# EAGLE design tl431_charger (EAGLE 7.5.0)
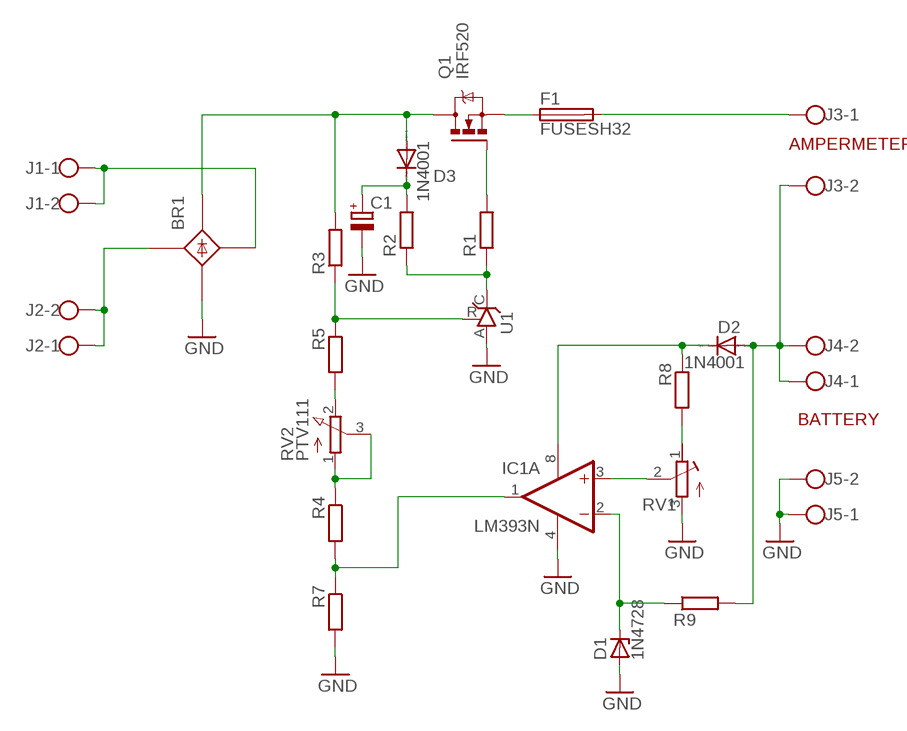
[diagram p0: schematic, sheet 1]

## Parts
BR1  B25A-  [B25A-]
C1  CPOL-EUE2.5-7  [E2,5-7]
D1  1N4728  [DO41Z10]
D2  1N4001  1N4004  [DO41-10]
D3  1N4001  1N4004  [DO41-10]
F1  FUSESH32  [SH32]
IC1  LM393N  [DIL08]
J1  W237-102  [W237-102]
J2  W237-102  [W237-102]
J3  W237-102  [W237-102]
J4  W237-102  [W237-102]
J5  W237-102  [W237-102]
Q1  IRF520  [TO220BV]
R1  R-EU_0207/10  [0207/10]
R2  R-EU_0207/10  [0207/10]
R3  R-EU_0207/10  [0207/10]
R4  R-EU_0207/10  [0207/10]
R5  R-EU_0207/10  [0207/10]
R7  R-EU_0207/10  [0207/10]
R8  R-EU_0207/10  [0207/10]
R9  R-EU_0207/10  [0207/10]
RV1  R-TRIMM-3386-F  [R-TRIMM-3386F]
RV2  PTV111  [PTV111]
U1  TL431CLP  [TO92-CLP]

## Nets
GND: BR1.-1(-) C1.- D1.A IC1.4(P:V-) J5.1 J5.2 R7.2 RV1.3(E) U1.A
N$1: IC1.1(A:OUT) R4.2 R7.1
N$2: Q1.G R1.2
N$3: F1.1A Q1.S
N$4: BR1.+1(+) D3.A Q1.D R3.2
N$5: C1.+ D3.C R2.2
N$6: R1.1 R2.1 U1.C
N$7: R5.2 RV2.2(E)
N$8: R3.1 R5.1 U1.R
N$9: R4.1 RV2.1(A) RV2.3(S)
N$10: IC1.3(A:+IN) RV1.2(S)
N$11: D1.C IC1.2(A:-IN) R9.1
N$12: BR1.AC1-(AC1) J2.1 J2.2
N$13: BR1.AC2-(AC2) J1.1 J1.2
N$14: R8.2 RV1.1(A)
N$15: D2.C IC1.8(P:V+) R8.1
N$16: D2.A J3.2 J4.1 J4.2 R9.2
N$17: F1.2A J3.1
Unconnected: BR1.+ BR1.- BR1.AC1 BR1.AC2 IC1.5(B:+IN) IC1.6(B:-IN) IC1.7(B:OUT)

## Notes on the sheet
- AMPERMETER
- BATTERY

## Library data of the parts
BR1 = rectifier:B25A-: RECTIFIER 25-A bridge
C1 = rcl:CPOL-EU: POLARIZED CAPACITOR, European symbol
D1 = diode:1N4728: Z DIODE
D2 D3 = diode:1N4004: DIODE
F1 = fuse:FUSE: Fuse; OC_FARNELL: unknown; OC_NEWARK: unknown
IC1 = linear:LM393: COMPARATOR
J1-J5 = con-wago-500:W237-102: WAGO SCREW CLAMP; MPN: 237-102; OC_FARNELL: unknown; OC_NEWARK: 70K9898
Q1 = transistor-power:IRF520: HEXFET Power MOSFET
R1-R5 R7-R9 = rcl:R-EU_: RESISTOR, European symbol
RV1 = rcl:R-TRIMM-3386-F
RV2 = pot:PTV111
U1 = v-reg:TL431CLP: VOLTAGE REGULATOR

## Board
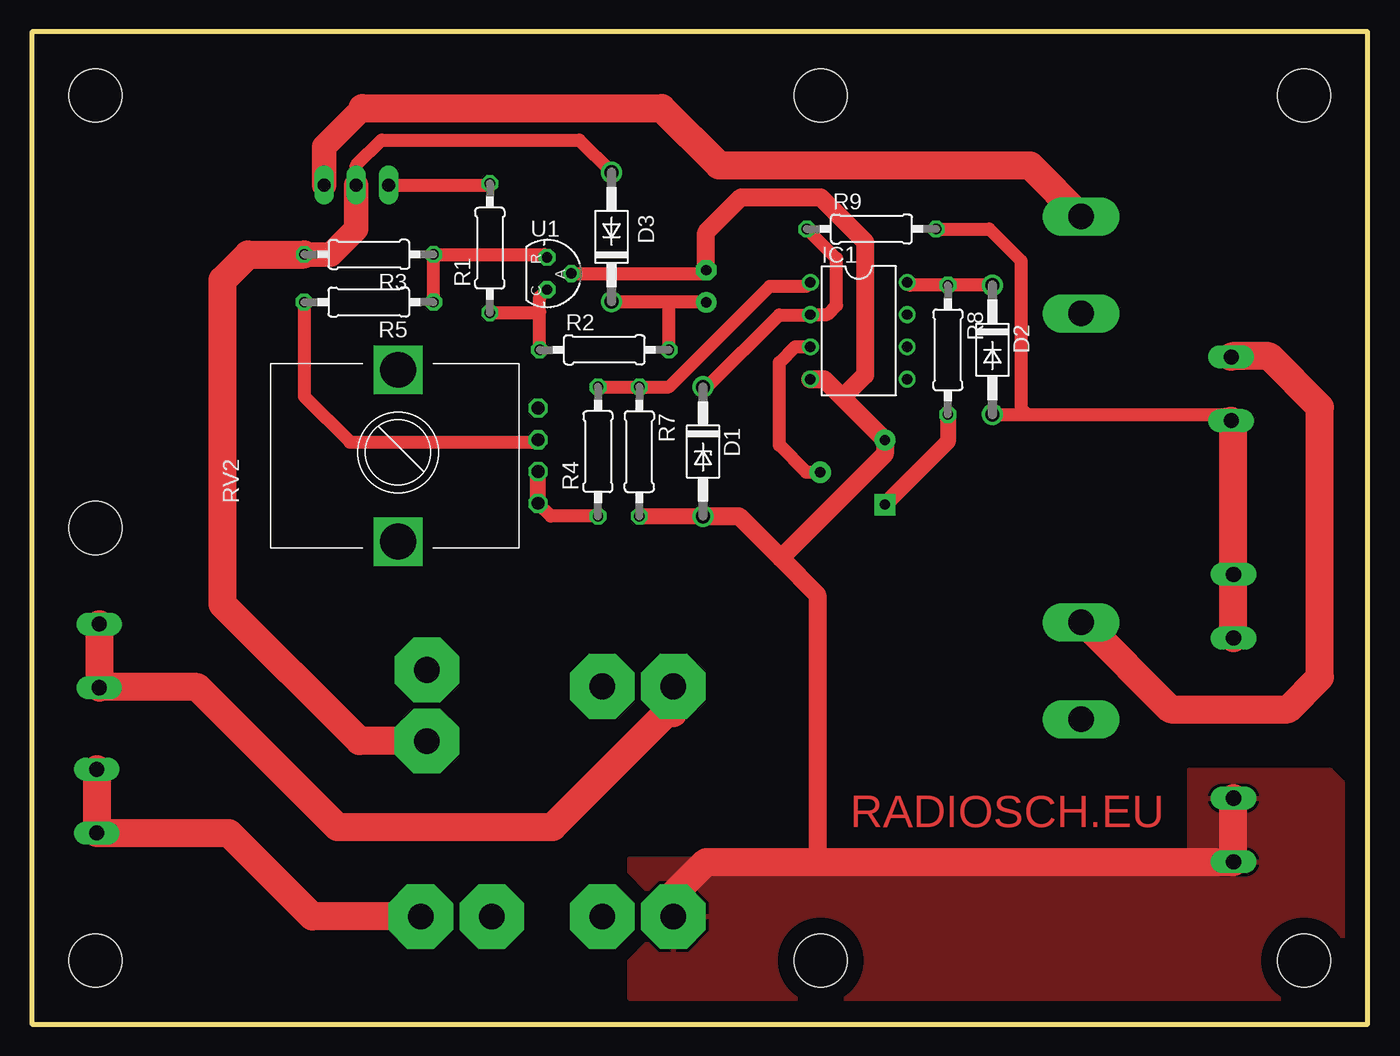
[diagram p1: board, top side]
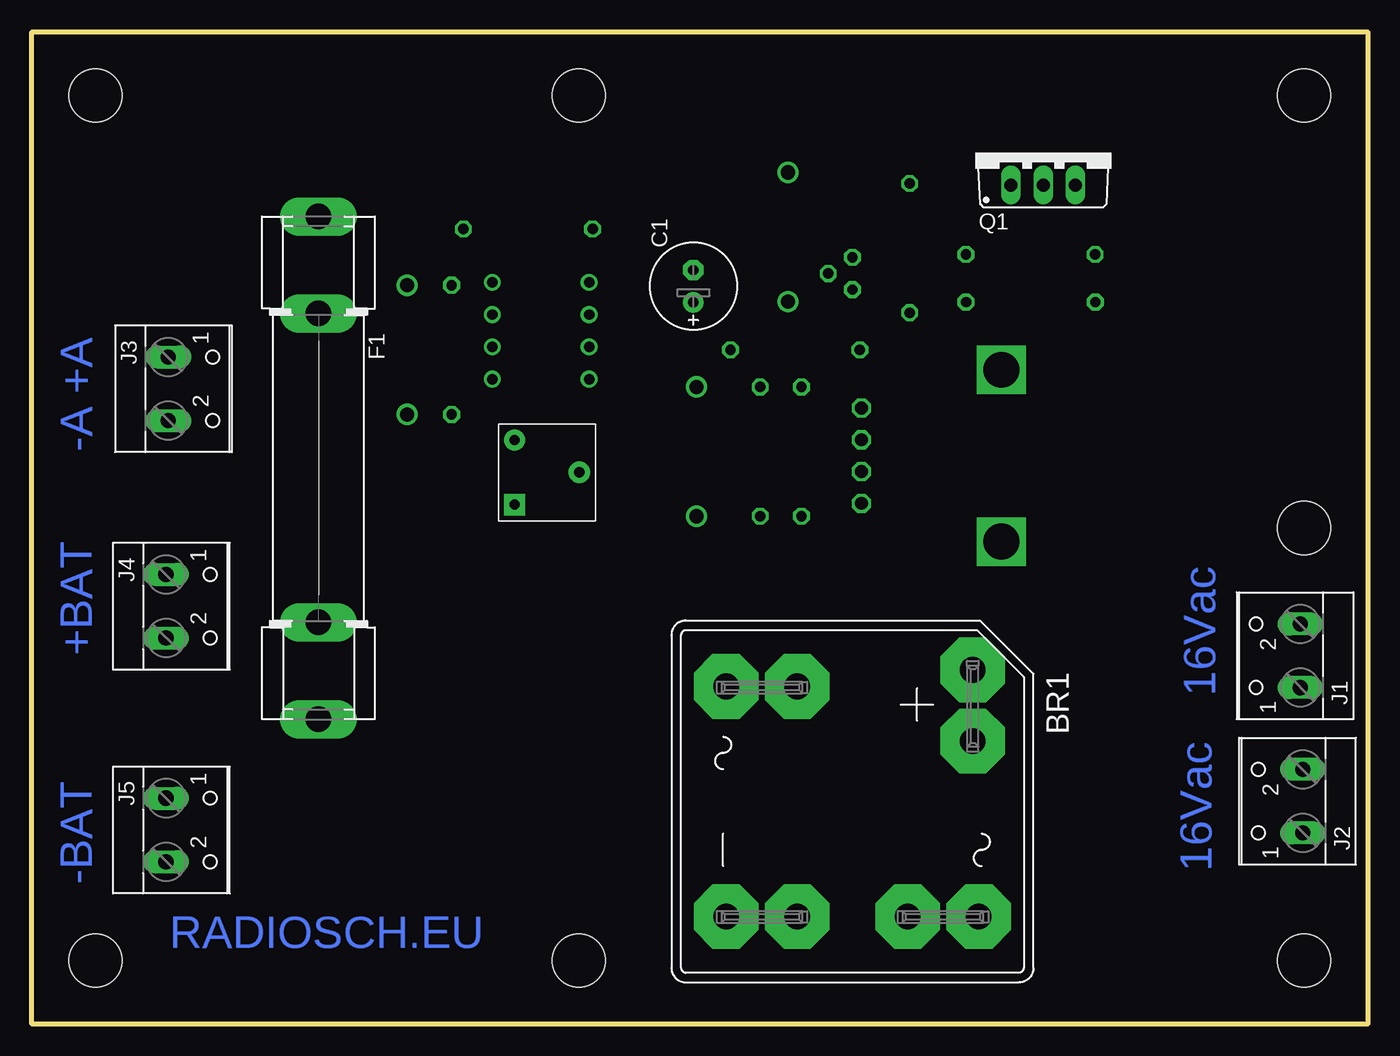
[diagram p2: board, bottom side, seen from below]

Size 105 x 78 mm. Coordinates in mm from the lower left corner, seen from the top.
Outline: 0,0 105,0 105,78 0,78 0,0
Copper layers (1*16): Top 0.035mm / dielectric 1.5mm / Bottom 0.035mm
Design rules "default": minimum track width 10mil, minimum drill 24mil, track to track 8mil, track to pad 8mil, pad to pad 8mil, via to via 8mil, smd to smd 8mil, copper to edge 40mil, drill to drill 8mil, minimum pad ring 10mil, minimum via ring 8mil, stop-mask expansion 4mil, vias tented up to drill 0mil, thermal gap 10mil
Holes 4.2 mm at 5,73 5,5 5,39 100,5 100,73 62,5 62,73

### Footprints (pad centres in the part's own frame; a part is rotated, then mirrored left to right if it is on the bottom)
B25A- = drill 2.007 pad 5.08 octagon: + -10.338,9.449; +1 -4.75,9.449; - 9.042,-4.343; -1 9.042,-9.931; AC1 9.042,4.343; AC1- 9.042,9.931; AC2 -9.042,-4.343; AC2- -9.042,-9.931
E2,5-7 = drill 0.813 pad 1.6: + -1.27,0 | drill 0.813 pad 1.6 octagon: - 1.27,0
DO41Z10 = drill 1.118: A 5.08,0; C -5.08,0
DO41-10 = drill 1.118: A 5.08,0; C -5.08,0
SH32 = drill 2.007 long: 1A -16.764,0; 1B -9.144,0; 2A 15.144,0; 2B 22.764,0
DIL08 = drill 0.813 pad 1.27: 1 -3.81,-3.81; 2 -1.27,-3.81; 3 1.27,-3.81; 4 3.81,-3.81; 5 3.81,3.81; 6 1.27,3.81; 7 -1.27,3.81; 8 -3.81,3.81
W237-102 = drill 1.194 long: 1 -2.5,-1.27; 2 2.5,-1.27
TO220BV = drill 1.016 long: D 0,-2.54; G -2.54,-2.54; S 2.54,-2.54
0207/10 = drill 0.813 octagon: 1 -5.08,0; 2 5.08,0
R-TRIMM-3386F = drill 0.8 pad 1.676 square: 1 0,0 | drill 0.8 pad 1.676: 2 5.08,2.54; 3 0,5.08
PTV111 = drill 1 octagon: 1 3,-11; 2 8,-11; 3 5.5,-11; 4 10.5,-11 | drill 2.8 square: P$1 0,0; P$2 13.5,0
TO92-CLP = drill 0.813 octagon: A 0,1.905; C 1.27,0; R -1.27,0

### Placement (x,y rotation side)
BR1  40.5,17.5 270 bottom
C1  53,58 90 bottom
D1  52.75,45 270 top
D2  75.5,53 270 top
D3  45.57,61.87 90 top
F1  82.47,46.72 270 bottom
IC1  65,54.5 270 top
J1  6.57,28.95 90 bottom
J2  6.38,17.52 90 bottom
J3  93,49.94 270 bottom
J4  93.18,32.85 270 bottom
J5  93.18,15.26 270 bottom
Q1  25.5,68.5 0 bottom
R1  36,61 90 top
R2  45,53 0 top
R3  26.5,60.5 180 top
R4  44.5,45 90 top
R5  26.49,56.75 180 top
R7  47.75,45 270 top
R8  72,53 270 top
R9  66,62.5 0 top
RV1  67.05,40.83 0 bottom
RV2  28.79,37.93 90 top
U1  40.5,59 270 top

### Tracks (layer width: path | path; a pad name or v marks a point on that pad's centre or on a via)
GND
  Top 1.016: U1.A 52.73,59 C1.-
  Top 1.27: R7.2 53.25,39.92
  Top 1.422: D1.A 53.25,39.92 55.58,39.92 58.88,36.62 | 58.88,36.62 61.75,33.75 61.75,13 61.5,12.75 | 58.88,36.62 67.05,44.8 RV1.3 63.73,49.23 | IC1.4 62.27,50.69 63.73,49.23 | C1.- 53,62.25 55.75,65 62,65 65.5,61.5 65.5,51 63.73,49.23
  Top 2.184: BR1.-1 50.43,10.18 53,12.75 61.5,12.75 J5.2 J5.1
  pour Top (isolate 1.27): 47,13 91,13 91,20 102,20 103,19 103,3 102,2 47,2
N$1
  Top 1.016: IC1.1 60.88,58 58,58 50.08,50.08 R7.1 R4.2
N$2
  Top 1.016: Q1.G 35.88,65.96 R1.2
N$3
  Top 1.93: Q1.S 22.96,68.96 26,72
  Top 2.184: 26,72 49.5,72 54,67.5 78.45,67.5 F1.1A
N$4
  Top 1.016: Q1.D 25.5,67.5 27.5,69.5 43.02,69.5 D3.A
  Top 1.93: Q1.D 25.5,62.5 23.5,60.5 R3.2
  Top 2.184: BR1.+1 25.75,22.25 15,33 15,58.5 17,60.5 R3.2
N$5
  Top 1.016: D3.C 50.25,56.79 | 50.25,56.79 52.94,56.79 C1.+ | R2.2 50.08,56.62 50.25,56.79
N$6
  Top 1.016: R2.1 39.92,56 | 39.92,56 39.92,57.15 U1.C | R1.1 39.84,55.92 39.92,56
N$7
  Top 1.016: R5.2 21.41,49.34 25,45.75 39.61,45.75 RV2.2
N$8
  Top 1.016: U1.R 40.27,60.5 R3.1 R5.1
N$9
  Top 1.016: R4.1 40.8,39.92 RV2.1
  Top 1.27: RV2.1 RV2.3
N$10
  Top 1.016: RV1.2 60.88,43.37 58.75,45.5 58.75,52 60,53.25 61.17,53.25 IC1.3
N$11
  Top 1.016: D1.C 53.08,50.08 58.75,55.75 61.17,55.75 IC1.2 62.52,55.77 63.25,56.5 63.25,60.17 R9.1
N$12
  Top 2.184: BR1.AC1- 22.04,8.46 15.5,15 5.13,15 J2.1 J2.2
N$13
  Top 2.184: J1.2 J1.1 5.35,26.5 13,26.5 24,15.5 40.93,15.5 50.43,25 | BR1.AC2- 50.43,25 | 50.43,25 50.43,24.43
N$14
  Top 1.27: R8.2 72,45.78 RV1.1
N$15
  Top 1.016: D2.C R8.1 69.04,58.08 IC1.8
N$16
  Top 1.016: D2.A 78.25,47.92 | 78.25,47.92 93.79,47.92 J3.2 | R9.2 75.25,62.5 77.75,60 77.75,48.42 78.25,47.92
  Top 2.184: J4.2 J4.1 94.45,47.26 J3.2
N$17
  Top 2.184: F1.2A 82.67,31.58 89.5,24.75 98.75,24.75 101.25,27.25 101.25,48.5 97.25,52.5 94.33,52.5 J3.1

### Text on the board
Top: RADIOSCH.EU
Bottom: -A +A | 16Vac | +BAT | 16Vac | -BAT | RADIOSCH.EU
